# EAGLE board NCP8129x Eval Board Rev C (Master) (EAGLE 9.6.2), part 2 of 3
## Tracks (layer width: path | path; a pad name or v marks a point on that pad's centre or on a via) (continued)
VIN  (via drill 0.15 pad 0.3) (continued)
  other vias: 37.23,60.63 37.63,60.63 38.03,60.63 38.43,60.63 38.83,60.63 39.23,60.63 39.63,60.63 40.03,60.63 37.43,60.98 37.83,60.98 38.23,60.98 38.63,60.98 39.03,60.98 39.43,60.98 39.83,60.98 37.23,61.33 37.63,61.33 38.03,61.33 38.43,61.33 38.83,61.33 39.23,61.33 39.63,61.33 40.03,61.33 37.43,61.68 37.83,61.68 38.23,61.68 38.63,61.68 39.03,61.68 39.43,61.68 39.83,61.68 37.23,62.03 37.63,62.03 38.03,62.03 38.43,62.03 38.83,62.03 39.23,62.03 39.63,62.03 40.03,62.03 37.43,62.38 37.83,62.38 38.23,62.38 38.63,62.38 39.03,62.38 39.43,62.38 39.83,62.38 37.23,62.73 37.63,62.73 38.03,62.73 38.43,62.73 38.83,62.73 39.23,62.73 39.63,62.73 40.03,62.73 37.43,63.08 37.83,63.08 38.23,63.08 38.63,63.08 39.03,63.08 39.43,63.08 39.83,63.08 37.23,63.43 37.63,63.43 38.03,63.43 38.43,63.43 38.83,63.43 39.23,63.43 39.63,63.43 40.03,63.43 37.43,63.78 37.83,63.78 38.23,63.78 38.63,63.78 39.03,63.78 39.43,63.78 39.83,63.78 65.38,31.13 65.78,31.13 66.18,31.13 66.58,31.13 66.98,31.13 67.38,31.13 67.78,31.13 65.18,31.43 65.58,31.43 65.98,31.43 66.38,31.43 66.78,31.43 67.18,31.43 67.58,31.43 67.98,31.43 65.38,31.73 65.78,31.73 66.18,31.73 66.58,31.73 66.98,31.73 67.38,31.73 67.78,31.73 65.18,32.03 65.58,32.03 65.98,32.03 66.38,32.03 66.78,32.03 67.18,32.03 67.58,32.03 67.98,32.03 65.38,32.33 65.78,32.33 66.18,32.33 66.58,32.33 66.98,32.33 67.38,32.33 67.78,32.33 65.18,32.63 65.58,32.63 65.98,32.63 66.38,32.63 66.78,32.63 67.18,32.63 67.58,32.63 67.98,32.63 65.38,32.93 65.78,32.93 66.18,32.93 66.58,32.93 66.98,32.93 67.38,32.93 67.78,32.93 65.18,33.23 65.58,33.23 65.98,33.23 66.38,33.23 66.78,33.23 67.18,33.23 67.58,33.23 67.98,33.23 67.78,33.53 67.38,33.53 66.98,33.53 66.58,33.53 66.18,33.53 65.78,33.53 65.38,33.53 65.18,33.83 65.58,33.83 65.98,33.83 66.38,33.83 66.78,33.83 67.18,33.83 67.58,33.83 67.98,33.83 37.43,60.28 37.03,60.28 37.83,60.28 38.23,60.28 38.63,60.28 39.03,60.28 39.43,60.28 39.83,60.28 37.23,59.93 37.63,59.93 38.03,59.93 38.43,59.93 38.83,59.93 39.23,59.93 39.63,59.93 36.83,59.93 37.03,59.58 37.43,59.58 37.83,59.58 38.23,59.58 38.63,59.58 39.03,59.58 39.43,59.58 39.83,59.58 36.83,59.23 37.23,59.23 37.63,59.23 38.03,59.23 38.43,59.23 38.83,59.23 39.23,59.23 39.63,59.23 39.83,58.88 39.43,58.88 39.03,58.88 38.63,58.88 38.23,58.88 37.83,58.88 37.43,58.88 37.03,58.88 36.63,58.88 36.63,59.58 36.43,59.23 36.23,58.88 36.43,58.53 36.03,58.53 36.83,58.53 37.23,58.53 37.63,58.53 38.03,58.53 38.43,58.53 38.83,58.53 39.23,58.53 39.63,58.53 40.03,58.53 35.78,49.83 35.38,49.83 34.98,49.83 34.58,49.83 34.18,49.83 33.78,49.83 33.38,49.83 32.98,49.83 32.58,49.83 32.18,49.83 35.58,49.53 35.18,49.53 34.78,49.53 34.38,49.53 33.98,49.53 33.58,49.53 33.18,49.53 32.38,49.53 32.78,49.53 31.98,49.53 35.98,49.53 32.18,49.23 32.58,49.23 32.98,49.23 33.38,49.23 33.78,49.23 34.18,49.23 34.58,49.23 34.98,49.23 35.38,49.23 35.78,49.23 31.98,48.93 32.38,48.93 32.78,48.93 33.18,48.93 33.58,48.93 33.98,48.93 34.38,48.93 34.78,48.93 35.18,48.93 35.58,48.93 35.98,48.93 32.18,48.63 32.58,48.63 32.98,48.63 33.38,48.63 33.78,48.63 34.18,48.63 34.58,48.63 34.98,48.63 35.38,48.63 35.78,48.63 31.98,48.33 32.38,48.33 32.78,48.33 33.18,48.33 33.58,48.33 33.98,48.33 34.38,48.33 34.78,48.33 35.18,48.33 35.58,48.33 35.98,48.33 35.78,48.03 35.38,48.03 34.98,48.03 34.58,48.03 34.18,48.03 32.18,48.03 32.58,48.03 32.98,48.03 33.38,48.03 33.78,48.03 45.08,49.83 44.68,49.83 44.28,49.83 43.88,49.83 43.48,49.83 43.08,49.83 42.68,49.83 42.28,49.83 41.88,49.83 41.48,49.83 44.88,49.53 44.48,49.53 44.08,49.53 43.68,49.53 43.28,49.53 42.88,49.53 42.48,49.53 41.68,49.53 42.08,49.53 41.28,49.53 45.28,49.53 41.48,49.23 41.88,49.23 42.28,49.23 42.68,49.23 43.08,49.23 43.48,49.23 43.88,49.23 44.28,49.23 44.68,49.23 45.08,49.23 41.28,48.93 41.68,48.93 42.08,48.93 42.48,48.93 42.88,48.93 43.28,48.93 43.68,48.93 44.08,48.93 44.48,48.93 44.88,48.93 45.28,48.93 41.48,48.63 41.88,48.63 42.28,48.63 42.68,48.63 43.08,48.63 43.48,48.63 43.88,48.63 44.28,48.63 44.68,48.63 45.08,48.63 41.28,48.33 41.68,48.33 42.08,48.33 42.48,48.33 42.88,48.33 43.28,48.33 43.68,48.33 44.08,48.33 44.48,48.33 44.88,48.33 45.28,48.33 45.08,48.03 44.68,48.03 44.28,48.03 43.88,48.03 43.48,48.03 41.48,48.03 41.88,48.03 42.28,48.03 42.68,48.03 43.08,48.03 36.13,56.48 35.73,56.48 35.33,56.48 35.93,56.18 35.53,56.18 36.13,55.88 35.73,55.88 35.33,55.88 35.93,55.58 35.53,55.58 36.13,55.28 35.73,55.28 35.33,55.28 41.93,56.48 41.53,56.48 41.13,56.48 41.73,56.18 41.33,56.18 41.93,55.88 41.53,55.88 41.13,55.88 41.73,55.58 41.33,55.58 41.93,55.28 41.53,55.28 41.13,55.28 35.53,54.98 35.33,54.68 35.53,54.38 35.33,54.08 35.53,53.78 35.33,53.48 35.13,54.98 35.13,54.38 35.13,53.78 34.93,53.48 34.73,53.78 34.93,54.08 34.93,54.68 34.73,54.38 34.53,54.08 34.33,53.78 34.53,53.48 34.53,54.68 34.33,54.38 34.13,54.08 33.93,53.78 34.13,53.48 34.13,54.68 33.93,54.38 33.73,54.08 33.53,53.78 33.73,53.48 33.53,54.38 33.73,54.68 41.73,54.98 41.93,54.68 41.73,54.38 41.93,54.08 41.73,53.78 41.93,53.48 42.13,53.78 42.13,54.38 42.13,54.98 42.33,54.68 42.53,54.38 42.33,54.08 42.53,53.78 42.33,53.48 42.73,54.68 43.13,54.68 43.53,54.68 42.93,54.38 43.33,54.38 43.73,54.38 42.73,54.08 43.13,54.08 43.53,54.08 42.93,53.78 43.33,53.78 43.73,53.78 42.73,53.48 43.13,53.48 43.53,53.48 36.63,56.63 37.43,56.63 38.23,56.63 39.03,56.63 40.63,56.63 37.03,56.23 37.83,56.23 38.63,56.23 40.23,56.23 36.63,55.83 37.43,55.83 38.23,55.83 39.83,55.83 40.63,55.83 37.03,55.43 37.83,55.43 39.43,55.43 40.23,55.43 36.63,55.03 37.43,55.03 39.03,55.03 39.83,55.03 40.63,55.03 37.03,54.63 36.23,54.63 38.63,54.63 39.43,54.63 40.23,54.63 41.03,54.63 36.63,54.23 38.23,54.23 39.03,54.23 39.83,54.23 40.63,54.23 36.23,53.83 37.83,53.83 38.63,53.83 39.43,53.83 40.23,53.83 41.03,53.83 41.43,53.43 40.63,53.43 39.83,53.43 39.03,53.43 38.23,53.43 37.43,53.43 35.83,53.43 35.43,53.03 34.63,53.03 33.83,53.03 35.03,52.63 34.23,52.63 41.03,51.43 41.83,51.43 42.63,51.43 43.43,51.43 40.23,51.43 39.43,51.43 38.63,51.43 37.83,51.43 43.03,51.03 42.23,51.03 41.43,51.03 40.63,51.03 39.83,51.03 39.03,51.03 38.23,51.03 37.43,51.03 37.83,50.63 38.63,50.63 39.43,50.63 40.23,50.63 41.03,50.63 41.83,50.63 42.63,50.63 43.43,50.63 44.23,50.63 37.03,50.63 37.43,50.23 38.23,50.23 39.03,50.23 39.83,50.23 40.63,50.23 41.43,50.23 42.23,50.23 43.03,50.23 43.83,50.23 44.63,50.23 36.63,50.23 35.83,50.23 35.03,50.23 34.23,50.23 33.43,50.23 32.63,50.23 37.03,49.83 37.83,49.83 38.63,49.83 39.43,49.83 40.23,49.83 41.03,49.83 40.63,49.43 39.83,49.43 39.03,49.43 38.23,49.43 37.43,49.43 36.63,49.43 36.23,49.83 37.03,49.03 37.83,49.03 38.63,49.03 39.43,49.03 40.23,49.03 36.63,48.63 37.43,48.63 38.23,48.63 39.03,48.63 39.83,48.63 40.63,48.63 37.03,48.23 37.83,48.23 38.63,48.23 39.43,48.23 40.23,48.23 36.63,47.83 37.43,47.83 38.23,47.83 39.03,47.83 39.83,47.83 40.63,47.83 40.63,44.63 41.43,44.63 42.23,44.63 43.03,44.63 43.83,44.63 44.63,44.63 39.83,44.63 39.03,44.63 38.23,44.63 37.43,44.63 36.63,44.63 35.83,44.63 35.03,44.63 34.23,44.63 33.43,44.63 33.03,44.23 33.83,44.23 34.63,44.23 35.43,44.23 36.23,44.23 37.03,44.23 37.83,44.23 38.63,44.23 39.43,44.23 40.23,44.23 41.03,44.23 41.83,44.23 42.63,44.23 43.43,44.23 44.23,44.23 45.03,44.23 32.63,43.83 33.43,43.83 34.23,43.83 35.03,43.83 35.83,43.83 36.63,43.83 37.43,43.83 38.23,43.83 39.03,43.83 39.83,43.83 40.63,43.83 41.43,43.83 42.23,43.83 43.03,43.83 43.83,43.83 44.63,43.83 32.23,43.43 33.03,43.43 33.83,43.43 34.63,43.43 35.43,43.43 36.23,43.43 37.03,43.43 37.83,43.43 38.63,43.43 39.43,43.43 40.23,43.43 45.03,43.43 44.23,43.43 43.43,43.43 42.63,43.43 41.83,43.43 41.03,43.43 32.63,43.03 33.43,43.03 34.23,43.03 35.03,43.03 35.83,43.03 36.63,43.03 37.43,43.03 38.23,43.03 39.03,43.03 44.63,43.03 43.83,43.03 43.03,43.03 42.23,43.03 41.43,43.03 40.63,43.03 39.83,43.03 45.03,42.63 44.23,42.63 43.43,42.63 42.63,42.63 41.83,42.63 41.03,42.63 40.23,42.63 39.43,42.63 38.63,42.63 37.83,42.63 32.23,42.63 33.03,42.63 33.83,42.63 34.63,42.63 35.43,42.63 36.23,42.63 37.03,42.63 32.63,42.23 33.43,42.23 34.23,42.23 35.03,42.23 35.83,42.23 36.63,42.23 37.43,42.23 38.23,42.23 39.03,42.23 39.83,42.23 40.63,42.23 41.43,42.23 42.23,42.23 43.03,42.23 43.83,42.23 44.63,42.23 45.03,41.83 44.23,41.83 43.43,41.83 42.63,41.83 41.83,41.83 41.03,41.83 40.23,41.83 39.43,41.83 38.63,41.83 37.83,41.83 37.03,41.83 36.23,41.83 35.43,41.83 34.63,41.83 33.83,41.83 33.03,41.83 32.23,41.83 32.63,41.43 33.43,41.43 34.23,41.43 35.03,41.43 35.83,41.43 36.63,41.43 37.43,41.43 38.23,41.43 39.03,41.43 39.83,41.43 40.63,41.43 41.43,41.43 42.23,41.43 43.03,41.43 43.83,41.43 44.63,41.43 45.03,41.03 44.23,41.03 43.43,41.03 42.63,41.03 41.83,41.03 41.03,41.03 40.23,41.03 39.43,41.03 38.63,41.03 37.83,41.03 37.03,41.03 36.23,41.03 35.43,41.03 34.63,41.03 33.83,41.03 33.03,41.03 32.23,41.03 32.63,40.63 33.43,40.63 34.23,40.63 35.03,40.63 35.83,40.63 36.63,40.63 37.43,40.63 38.23,40.63 39.03,40.63 44.63,40.63 43.83,40.63 43.03,40.63 42.23,40.63 41.43,40.63 40.63,40.63 39.83,40.63 45.03,40.23 44.23,40.23 43.43,40.23 42.63,40.23 41.83,40.23 41.03,40.23 40.23,40.23 39.43,40.23 38.63,40.23 37.83,40.23 32.23,40.23 33.03,40.23 33.83,40.23 34.63,40.23 35.43,40.23 36.23,40.23 37.03,40.23 32.63,39.83 33.43,39.83 34.23,39.83 35.03,39.83 35.83,39.83 36.63,39.83 37.43,39.83 38.23,39.83 39.03,39.83 39.83,39.83 40.63,39.83 41.43,39.83 42.23,39.83 43.03,39.83 43.83,39.83 44.63,39.83 45.03,39.43 44.23,39.43 43.43,39.43 42.63,39.43 41.83,39.43 41.03,39.43 40.23,39.43 39.43,39.43 38.63,39.43 37.83,39.43 37.03,39.43 36.23,39.43 35.43,39.43 34.63,39.43 33.83,39.43 33.03,39.43 32.23,39.43 32.63,39.03 33.43,39.03 34.23,39.03 35.03,39.03 35.83,39.03 36.63,39.03 37.43,39.03 38.23,39.03 39.03,39.03 39.83,39.03 40.63,39.03 41.43,39.03 42.23,39.03 43.03,39.03 43.83,39.03 44.63,39.03 45.03,38.63 44.23,38.63 43.43,38.63 42.63,38.63 41.83,38.63 41.03,38.63 40.23,38.63 39.43,38.63 38.63,38.63 37.83,38.63 37.03,38.63 36.23,38.63 35.43,38.63 34.63,38.63 33.83,38.63 33.03,38.63 32.23,38.63 32.63,38.23 33.43,38.23 34.23,38.23 35.03,38.23 35.83,38.23 36.63,38.23 37.43,38.23 38.23,38.23 39.03,38.23 44.63,38.23 43.83,38.23 43.03,38.23 42.23,38.23 41.43,38.23 40.63,38.23 39.83,38.23 45.03,37.83 44.23,37.83 43.43,37.83 42.63,37.83 41.83,37.83 41.03,37.83 40.23,37.83 39.43,37.83 38.63,37.83 37.83,37.83 32.23,37.83 33.03,37.83 33.83,37.83 34.63,37.83 35.43,37.83 36.23,37.83 37.03,37.83 32.63,37.43 33.43,37.43 34.23,37.43 35.03,37.43 35.83,37.43 36.63,37.43 37.43,37.43 38.23,37.43 39.03,37.43 39.83,37.43 40.63,37.43 41.43,37.43 42.23,37.43 43.03,37.43 43.83,37.43 44.63,37.43 45.03,37.03 44.23,37.03 43.43,37.03 42.63,37.03 41.83,37.03 41.03,37.03 40.23,37.03 39.43,37.03 38.63,37.03 37.83,37.03 37.03,37.03 36.23,37.03 35.43,37.03 34.63,37.03 33.83,37.03 33.03,37.03 32.23,37.03 32.63,36.63 33.43,36.63 34.23,36.63 35.03,36.63 35.83,36.63 36.63,36.63 37.43,36.63 38.23,36.63 39.03,36.63 39.83,36.63 40.63,36.63 41.43,36.63 42.23,36.63 43.03,36.63 43.83,36.63 44.63,36.63 45.03,36.23 44.23,36.23 43.43,36.23 42.63,36.23 41.83,36.23 41.03,36.23 40.23,36.23 39.43,36.23 38.63,36.23 37.83,36.23 37.03,36.23 36.23,36.23 35.43,36.23 34.63,36.23 33.83,36.23 33.03,36.23 32.23,36.23 32.63,35.83 33.43,35.83 34.23,35.83 35.03,35.83 35.83,35.83 36.63,35.83 37.43,35.83 38.23,35.83 39.03,35.83 44.63,35.83 43.83,35.83 43.03,35.83 42.23,35.83 41.43,35.83 40.63,35.83 39.83,35.83 45.03,35.43 44.23,35.43 43.43,35.43 42.63,35.43 41.83,35.43 41.03,35.43 40.23,35.43 39.43,35.43 38.63,35.43 37.83,35.43 32.23,35.43 33.03,35.43 33.83,35.43 34.63,35.43 35.43,35.43 36.23,35.43 37.03,35.43 32.63,35.03 33.43,35.03 34.23,35.03 35.03,35.03 35.83,35.03 36.63,35.03 37.43,35.03 38.23,35.03 39.03,35.03 39.83,35.03 40.63,35.03 41.43,35.03 42.23,35.03 43.03,35.03 43.83,35.03 44.63,35.03 45.03,34.63 44.23,34.63 43.43,34.63 42.63,34.63 41.83,34.63 41.03,34.63 40.23,34.63 39.43,34.63 38.63,34.63 37.83,34.63 37.03,34.63 36.23,34.63 35.43,34.63 34.63,34.63 33.83,34.63 33.03,34.63 32.23,34.63 32.63,34.23 33.43,34.23 34.23,34.23 35.03,34.23 35.83,34.23 36.63,34.23 37.43,34.23 38.23,34.23 39.03,34.23 39.83,34.23 40.63,34.23 41.43,34.23 42.23,34.23 43.03,34.23 43.83,34.23 44.63,34.23 45.03,33.83 44.23,33.83 43.43,33.83 42.63,33.83 41.83,33.83 41.03,33.83 40.23,33.83 39.43,33.83 38.63,33.83 37.83,33.83 37.03,33.83 36.23,33.83 35.43,33.83 34.63,33.83 33.83,33.83 33.03,33.83 32.23,33.83 32.63,33.43 33.43,33.43 34.23,33.43 35.03,33.43 35.83,33.43 36.63,33.43 37.43,33.43 38.23,33.43 39.03,33.43 44.63,33.43 43.83,33.43 43.03,33.43 42.23,33.43 41.43,33.43 40.63,33.43 39.83,33.43 45.03,33.03 44.23,33.03 43.43,33.03 42.63,33.03 41.83,33.03 41.03,33.03 40.23,33.03 39.43,33.03 38.63,33.03 37.83,33.03 32.23,33.03 33.03,33.03 33.83,33.03 34.63,33.03 35.43,33.03 36.23,33.03 37.03,33.03 32.63,32.63 33.43,32.63 34.23,32.63 35.03,32.63 35.83,32.63 36.63,32.63 37.43,32.63 38.23,32.63 39.03,32.63 39.83,32.63 40.63,32.63 41.43,32.63 42.23,32.63 43.03,32.63 43.83,32.63 44.63,32.63 45.03,32.23 44.23,32.23 43.43,32.23 42.63,32.23 41.83,32.23 41.03,32.23 40.23,32.23 39.43,32.23 38.63,32.23 37.83,32.23 37.03,32.23 36.23,32.23 35.43,32.23 34.63,32.23 33.83,32.23 33.03,32.23 32.23,32.23 32.63,31.83 33.43,31.83 34.23,31.83 35.03,31.83 35.83,31.83 36.63,31.83 37.43,31.83 38.23,31.83 39.03,31.83 39.83,31.83 40.63,31.83 41.43,31.83 42.23,31.83 43.03,31.83 43.83,31.83 44.63,31.83 45.03,31.43 44.23,31.43 43.43,31.43 42.63,31.43 41.83,31.43 41.03,31.43 40.23,31.43 39.43,31.43 38.63,31.43 37.83,31.43 37.03,31.43 36.23,31.43 35.43,31.43 34.63,31.43 33.83,31.43 33.03,31.43 32.23,31.43 32.63,31.03 33.43,31.03 34.23,31.03 35.03,31.03 35.83,31.03 36.63,31.03 37.43,31.03 38.23,31.03 39.03,31.03 44.63,31.03 43.83,31.03 43.03,31.03 42.23,31.03 41.43,31.03 40.63,31.03 39.83,31.03 45.03,30.63 44.23,30.63 43.43,30.63 42.63,30.63 41.83,30.63 41.03,30.63 40.23,30.63 39.43,30.63 38.63,30.63 37.83,30.63 32.23,30.63 33.03,30.63 33.83,30.63 34.63,30.63 35.43,30.63 36.23,30.63 37.03,30.63 32.63,30.23 33.43,30.23 34.23,30.23 35.03,30.23 35.83,30.23 36.63,30.23 37.43,30.23 38.23,30.23 39.03,30.23 39.83,30.23 40.63,30.23 41.43,30.23 42.23,30.23 43.03,30.23 43.83,30.23 44.63,30.23 45.03,29.83 44.23,29.83 43.43,29.83 42.63,29.83 41.83,29.83 41.03,29.83 40.23,29.83 39.43,29.83 38.63,29.83 37.83,29.83 37.03,29.83 36.23,29.83 35.43,29.83 34.63,29.83 33.83,29.83 33.03,29.83 32.23,29.83 32.63,29.43 33.43,29.43 34.23,29.43 35.03,29.43 35.83,29.43 36.63,29.43 37.43,29.43 38.23,29.43 39.03,29.43 39.83,29.43 40.63,29.43 41.43,29.43 42.23,29.43 43.03,29.43 43.83,29.43 44.63,29.43 45.03,29.03 44.23,29.03 43.43,29.03 42.63,29.03 41.83,29.03 41.03,29.03 40.23,29.03 39.43,29.03 38.63,29.03 37.83,29.03 37.03,29.03 36.23,29.03 35.43,29.03 34.63,29.03 33.83,29.03 33.03,29.03 32.23,29.03 32.63,28.63 33.43,28.63 34.23,28.63 35.03,28.63 35.83,28.63 36.63,28.63 37.43,28.63 38.23,28.63 39.03,28.63 44.63,28.63 43.83,28.63 43.03,28.63 42.23,28.63 41.43,28.63 40.63,28.63 39.83,28.63 45.03,28.23 44.23,28.23 43.43,28.23 42.63,28.23 41.83,28.23 41.03,28.23 40.23,28.23 39.43,28.23 38.63,28.23 37.83,28.23 32.23,28.23 33.03,28.23 33.83,28.23 34.63,28.23 35.43,28.23 36.23,28.23 37.03,28.23 32.63,27.83 33.43,27.83 34.23,27.83 35.03,27.83 35.83,27.83 36.63,27.83 37.43,27.83 38.23,27.83 39.03,27.83 39.83,27.83 40.63,27.83 41.43,27.83 42.23,27.83 43.03,27.83 43.83,27.83 44.63,27.83 45.03,27.43 44.23,27.43 43.43,27.43 42.63,27.43 41.83,27.43 41.03,27.43 40.23,27.43 39.43,27.43 38.63,27.43 37.83,27.43 37.03,27.43 36.23,27.43 35.43,27.43 34.63,27.43 33.83,27.43 33.03,27.43 32.23,27.43 32.63,27.03 33.43,27.03 34.23,27.03 35.03,27.03 35.83,27.03 36.63,27.03 37.43,27.03 38.23,27.03 39.03,27.03 39.83,27.03 40.63,27.03 41.43,27.03 42.23,27.03 43.03,27.03 43.83,27.03 44.63,27.03 45.03,26.63 44.23,26.63 43.43,26.63 42.63,26.63 41.83,26.63 41.03,26.63 40.23,26.63 39.43,26.63 38.63,26.63 37.83,26.63 37.03,26.63 36.23,26.63 35.43,26.63 34.63,26.63 33.83,26.63 33.03,26.63 32.23,26.63 32.63,26.23 33.43,26.23 34.23,26.23 35.03,26.23 35.83,26.23 36.63,26.23 37.43,26.23 38.23,26.23 39.03,26.23 44.63,26.23 43.83,26.23 43.03,26.23 42.23,26.23 41.43,26.23 40.63,26.23 39.83,26.23 45.03,25.83 44.23,25.83 43.43,25.83 42.63,25.83 41.83,25.83 41.03,25.83 40.23,25.83 39.43,25.83 38.63,25.83 37.83,25.83 32.23,25.83 33.03,25.83 33.83,25.83 34.63,25.83 35.43,25.83 36.23,25.83 37.03,25.83 32.63,25.43 33.43,25.43 34.23,25.43 35.03,25.43 35.83,25.43 36.63,25.43 37.43,25.43 38.23,25.43 39.03,25.43 39.83,25.43 40.63,25.43 41.43,25.43 42.23,25.43 43.03,25.43 43.83,25.43 44.63,25.43 45.03,25.03 44.23,25.03 43.43,25.03 42.63,25.03 41.83,25.03 41.03,25.03 40.23,25.03 39.43,25.03 38.63,25.03 37.83,25.03 37.03,25.03 36.23,25.03 35.43,25.03 34.63,25.03 33.83,25.03 33.03,25.03 33.43,24.63 34.23,24.63 35.03,24.63 35.83,24.63 36.63,24.63 37.43,24.63 38.23,24.63 39.03,24.63 39.83,24.63 40.63,24.63 41.43,24.63 42.23,24.63 43.03,24.63 43.83,24.63 44.63,24.63 45.03,24.23 44.23,24.23 43.43,24.23 42.63,24.23 41.83,24.23 41.03,24.23 40.23,24.23 39.43,24.23 38.63,24.23 37.83,24.23 37.03,24.23 36.23,24.23 35.43,24.23 34.63,24.23 33.83,24.23 45.43,39.83 45.43,39.03 45.43,38.23 45.43,37.43 45.43,36.63 45.43,35.83 45.43,35.03 45.43,34.23 45.43,33.43 45.43,32.63 45.43,31.83 45.43,31.03 45.83,31.43 45.83,32.23 45.83,33.03 45.83,33.83 45.83,34.63 45.83,35.43 45.83,36.23 45.83,37.03 45.83,37.83 45.83,38.63 45.83,39.43 46.23,39.03 46.23,38.23 46.23,37.43 46.23,36.63 46.23,35.83 46.23,35.03 46.23,34.23 46.23,33.43 46.23,32.63 46.23,31.83 46.63,32.23 46.63,33.03 46.63,33.83 46.63,34.63 46.63,35.43 46.63,36.23 46.63,37.03 46.63,37.83 46.63,38.63 47.03,38.23 47.03,37.43 47.03,36.63 47.03,35.83 47.03,35.03 47.03,34.23 47.03,33.43 47.03,32.63 47.43,33.03 47.43,33.83 47.43,34.63 47.43,35.43 47.43,36.23 47.43,37.03 47.43,37.83 47.83,36.63 47.83,37.43 47.83,35.83 47.83,35.03 47.83,34.23 47.83,33.43 48.23,33.83 48.23,34.63 48.23,35.43 48.23,36.23 48.23,37.03 48.23,33.03 47.83,32.63 48.23,32.23 47.83,31.83 48.23,31.43 47.83,31.03 48.23,30.63 47.83,30.23 48.23,29.83 47.83,29.43 48.23,29.03 47.83,28.63 48.23,28.23 47.83,27.83 48.23,27.43 47.83,27.03 47.43,32.23 47.43,31.43 47.43,30.63 47.43,29.83 47.43,29.03 47.43,28.23 47.43,27.43 47.03,27.83 47.03,28.63 47.03,29.43 47.03,30.23 47.03,31.03 47.03,31.83 46.63,31.43 46.63,30.63 46.63,29.83 46.63,29.03 46.63,28.23 46.23,29.43 46.23,30.23 46.23,31.03 45.83,30.63 45.83,29.83 46.23,28.63 45.83,29.03 45.43,30.23 45.43,29.43 45.43,28.63 45.83,28.23 46.23,27.83 46.63,27.43 47.03,27.03 47.43,26.63 47.83,26.23 48.23,26.63 45.43,27.83 45.83,27.43 46.23,27.03 46.63,26.63 47.03,26.23 47.43,25.83 47.83,25.43 48.23,25.83 48.23,25.03 45.43,27.03 45.83,26.63 46.23,26.23 46.63,25.83 47.03,25.43 47.43,25.03 47.83,24.63 48.23,24.23 45.43,26.23 45.83,25.83 46.23,25.43 46.63,25.03 47.03,24.63 47.43,24.23 47.83,23.83 48.23,23.43 45.43,25.43 45.83,25.03 46.23,24.63 46.63,24.23 47.03,23.83 47.43,23.43 47.83,23.03 48.23,22.63 45.43,24.63 45.83,24.23 46.23,23.83 46.63,23.43 47.03,23.03 47.43,22.63 47.83,22.23 48.23,21.83 48.63,23.83 49.43,23.83 50.23,23.83 51.03,23.83 51.83,23.83 52.63,23.83 53.43,23.83 54.23,23.83 55.03,23.83 55.83,23.83 56.63,23.83 57.43,23.83 58.23,23.83 59.03,23.83 59.83,23.83 60.63,23.83 61.43,23.83 61.03,23.43 60.23,23.43 59.43,23.43 58.63,23.43 57.83,23.43 57.03,23.43 56.23,23.43 55.43,23.43 54.63,23.43 53.83,23.43 53.03,23.43 52.23,23.43 51.43,23.43 49.03,23.43 49.83,23.43 50.63,23.43 48.63,23.03 49.43,23.03 50.23,23.03 51.03,23.03 51.83,23.03 52.63,23.03 53.43,23.03 54.23,23.03 55.03,23.03 55.83,23.03 60.63,23.03 59.83,23.03 59.03,23.03 58.23,23.03 57.43,23.03 56.63,23.03 49.03,22.63 49.83,22.63 50.63,22.63 51.43,22.63 52.23,22.63 53.03,22.63 53.83,22.63 54.63,22.63 55.43,22.63 56.23,22.63 57.03,22.63 57.83,22.63 58.63,22.63 59.43,22.63 60.23,22.63 61.03,22.63 60.63,22.23 60.23,21.83 34.23,23.83 35.03,23.83 35.83,23.83 36.63,23.83 37.43,23.83 38.23,23.83 39.03,23.83 39.83,23.83 40.63,23.83 41.43,23.83 42.23,23.83 43.03,23.83 43.83,23.83 44.63,23.83 45.43,23.83 34.63,23.43 35.43,23.43 36.23,23.43 37.03,23.43 37.83,23.43 38.63,23.43 39.43,23.43 40.23,23.43 41.03,23.43 41.83,23.43 42.63,23.43 43.43,23.43 44.23,23.43 45.03,23.43 45.83,23.43 35.03,23.03 35.83,23.03 36.63,23.03 37.43,23.03 38.23,23.03 39.03,23.03 39.83,23.03 40.63,23.03 41.43,23.03 42.23,23.03 43.03,23.03 43.83,23.03 44.63,23.03 45.43,23.03 46.23,23.03 35.43,22.63 36.23,22.63 37.03,22.63 37.83,22.63 38.63,22.63 39.43,22.63 40.23,22.63 41.03,22.63 41.83,22.63 42.63,22.63 43.43,22.63 44.23,22.63 45.03,22.63 45.83,22.63 46.63,22.63 35.83,22.23 36.63,22.23 37.43,22.23 38.23,22.23 39.03,22.23 39.83,22.23 40.63,22.23 41.43,22.23 42.23,22.23 43.03,22.23 43.83,22.23 44.63,22.23 45.43,22.23 46.23,22.23 47.03,22.23 36.23,21.83 37.03,21.83 37.83,21.83 38.63,21.83 39.43,21.83 40.23,21.83 41.03,21.83 41.83,21.83 42.63,21.83 43.43,21.83 44.23,21.83 45.03,21.83 45.83,21.83 46.63,21.83 47.43,21.83 48.63,22.23 49.03,21.83 49.43,22.23 49.83,21.83 50.23,22.23 50.63,21.83 51.03,22.23 51.43,21.83 51.83,22.23 52.23,21.83 52.63,22.23 53.03,21.83 53.43,22.23 53.83,21.83 54.23,22.23 54.63,21.83 55.03,22.23 55.43,21.83 55.83,22.23 56.23,21.83 56.63,22.23 57.03,21.83 57.43,22.23 57.83,21.83 58.23,22.23 58.63,21.83 59.03,22.23 59.43,21.83 59.83,22.23 36.63,21.43 37.43,21.43 38.23,21.43 39.03,21.43 39.83,21.43 40.63,21.43 41.43,21.43 42.23,21.43 43.03,21.43 59.83,21.43 59.03,21.43 58.23,21.43 57.43,21.43 56.63,21.43 55.83,21.43 55.03,21.43 54.23,21.43 53.43,21.43 52.63,21.43 51.83,21.43 51.03,21.43 50.23,21.43 49.43,21.43 48.63,21.43 47.83,21.43 47.03,21.43 46.23,21.43 45.43,21.43 44.63,21.43 43.83,21.43 37.03,21.03 37.83,21.03 38.63,21.03 39.43,21.03 40.23,21.03 41.03,21.03 41.83,21.03 42.63,21.03 43.43,21.03 44.23,21.03 45.03,21.03 45.83,21.03 46.63,21.03 47.43,21.03 48.23,21.03 49.03,21.03 49.83,21.03 50.63,21.03 51.43,21.03 52.23,21.03 53.03,21.03 53.83,21.03 54.63,21.03 55.43,21.03 56.23,21.03 57.03,21.03 57.83,21.03 58.63,21.03 59.43,21.03 37.43,20.63 38.23,20.63 39.03,20.63 39.83,20.63 40.63,20.63 41.43,20.63 42.23,20.63 43.03,20.63 43.83,20.63 44.63,20.63 45.43,20.63 46.23,20.63 47.03,20.63 47.83,20.63 48.63,20.63 49.43,20.63 50.23,20.63 51.03,20.63 51.83,20.63 52.63,20.63 53.43,20.63 54.23,20.63 55.03,20.63 55.83,20.63 56.63,20.63 57.43,20.63 58.23,20.63 59.03,20.63 37.83,20.23 38.63,20.23 39.43,20.23 40.23,20.23 41.03,20.23 41.83,20.23 42.63,20.23 43.43,20.23 44.23,20.23 45.03,20.23 45.83,20.23 46.63,20.23 47.43,20.23 48.23,20.23 49.03,20.23 49.83,20.23 50.63,20.23 51.43,20.23 52.23,20.23 53.03,20.23 53.83,20.23 54.63,20.23 55.43,20.23 56.23,20.23 57.03,20.23 57.83,20.23 58.63,20.23 38.23,19.83 39.03,19.83 39.83,19.83 40.63,19.83 41.43,19.83 42.23,19.83 43.03,19.83 43.83,19.83 44.63,19.83 45.43,19.83 46.23,19.83 47.03,19.83 47.83,19.83 48.63,19.83 49.43,19.83 50.23,19.83 51.03,19.83 51.83,19.83 52.63,19.83 53.43,19.83 54.23,19.83 55.03,19.83 55.83,19.83 56.63,19.83 57.43,19.83 58.23,19.83 38.63,19.43 39.43,19.43 40.23,19.43 41.03,19.43 41.83,19.43 42.63,19.43 43.43,19.43 44.23,19.43 45.03,19.43 45.83,19.43 46.63,19.43 47.43,19.43 48.23,19.43 49.03,19.43 49.83,19.43 50.63,19.43 51.43,19.43 52.23,19.43 53.03,19.43 53.83,19.43 54.63,19.43 55.43,19.43 56.23,19.43 57.03,19.43 57.83,19.43 39.03,19.03 39.83,19.03 40.63,19.03 41.43,19.03 42.23,19.03 43.03,19.03 43.83,19.03 44.63,19.03 45.43,19.03 46.23,19.03 47.03,19.03 47.83,19.03 48.63,19.03 49.43,19.03 50.23,19.03 51.03,19.03 51.83,19.03 52.63,19.03 53.43,19.03 54.23,19.03 55.03,19.03 55.83,19.03 56.63,19.03 57.43,19.03 57.03,18.63 56.23,18.63 55.43,18.63 54.63,18.63 53.83,18.63 53.03,18.63 52.23,18.63 51.43,18.63 50.63,18.63 49.83,18.63 49.03,18.63 48.23,18.63 47.43,18.63 46.63,18.63 39.43,18.63 40.23,18.63 41.03,18.63 41.83,18.63 42.63,18.63 43.43,18.63 44.23,18.63 45.03,18.63 45.83,18.63 39.83,18.23 40.63,18.23 41.43,18.23 42.23,18.23 43.03,18.23 43.83,18.23 44.63,18.23 45.43,18.23 46.23,18.23 47.03,18.23 47.83,18.23 48.63,18.23 49.43,18.23 50.23,18.23 51.03,18.23 51.83,18.23 52.63,18.23 53.43,18.23 54.23,18.23 55.03,18.23 55.83,18.23 56.63,18.23 56.23,17.83 55.43,17.83 54.63,17.83 53.83,17.83 53.03,17.83 52.23,17.83 51.43,17.83 50.63,17.83 49.83,17.83 49.03,17.83 48.23,17.83 47.43,17.83 46.63,17.83 45.83,17.83 45.03,17.83 44.23,17.83 43.43,17.83 42.63,17.83 41.83,17.83 41.03,17.83 40.23,17.83 40.63,17.43 41.43,17.43 42.23,17.43 43.03,17.43 43.83,17.43 44.63,17.43 45.43,17.43 46.23,17.43 47.03,17.43 47.83,17.43 48.63,17.43 49.43,17.43 50.23,17.43 51.03,17.43 51.83,17.43 52.63,17.43 53.43,17.43 54.23,17.43 55.03,17.43 55.83,17.43 55.43,17.03 54.63,17.03 53.83,17.03 53.03,17.03 52.23,17.03 51.43,17.03 50.63,17.03 49.83,17.03 49.03,17.03 48.23,17.03 47.43,17.03 46.63,17.03 45.83,17.03 45.03,17.03 44.23,17.03 43.43,17.03 42.63,17.03 41.83,17.03 41.03,17.03 41.43,16.63 42.23,16.63 43.03,16.63 43.83,16.63 44.63,16.63 45.43,16.63 46.23,16.63 47.03,16.63 47.83,16.63 48.63,16.63 49.43,16.63 50.23,16.63 51.03,16.63 51.83,16.63 52.63,16.63 53.43,16.63 54.23,16.63 55.03,16.63 54.63,16.23 53.83,16.23 53.03,16.23 52.23,16.23 51.43,16.23 50.63,16.23 49.83,16.23 49.03,16.23 48.23,16.23 47.43,16.23 46.63,16.23 45.83,16.23 45.03,16.23 44.23,16.23 43.43,16.23 42.63,16.23 41.83,16.23 42.23,15.83 43.03,15.83 43.83,15.83 44.63,15.83 45.43,15.83 46.23,15.83 47.03,15.83 47.83,15.83 48.63,15.83 49.43,15.83 50.23,15.83 51.03,15.83 51.83,15.83 52.63,15.83 53.43,15.83 54.23,15.83 53.83,15.43 53.03,15.43 52.23,15.43 51.43,15.43 50.63,15.43 49.83,15.43 49.03,15.43 48.23,15.43 47.43,15.43 46.63,15.43 45.83,15.43 45.03,15.43 44.23,15.43 43.43,15.43 42.63,15.43 43.03,15.03 43.83,15.03 44.63,15.03 45.43,15.03 46.23,15.03 47.03,15.03 47.83,15.03 48.63,15.03 49.43,15.03 50.23,15.03 51.03,15.03 51.83,15.03 52.63,15.03 53.43,15.03 53.83,14.63 53.03,14.63 52.23,14.63 51.43,14.63 50.63,14.63 49.83,14.63 49.03,14.63 48.23,14.63 47.43,14.63 46.63,14.63 45.83,14.63 45.03,14.63 44.23,14.63 43.43,14.63 43.83,14.23 44.63,14.23 45.43,14.23 46.23,14.23 47.03,14.23 47.83,14.23 48.63,14.23 49.43,14.23 50.23,14.23 51.03,14.23 51.83,14.23 52.63,14.23 53.43,14.23 53.83,13.83 53.43,13.43 53.83,13.03 53.43,12.63 53.83,12.23 53.43,11.83 53.83,11.43 53.43,11.03 53.83,10.63 53.43,10.23 53.83,9.83 53.43,9.43 53.83,9.03 53.43,8.63 53.83,8.23 53.43,7.83 53.83,7.43 53.43,7.03 53.83,6.63 53.43,6.23 53.83,5.83 53.43,5.43 53.83,5.03 53.43,4.63 53.83,4.23 53.43,3.83 53.83,3.43 53.43,3.03 53.03,3.43 52.63,3.03 52.23,3.43 51.83,3.03 51.43,3.43 51.03,3.03 50.63,3.43 50.23,3.03 49.83,3.43 49.43,3.03 49.03,3.43 48.63,3.03 48.23,3.43 47.83,3.03 47.43,3.43 47.03,3.03 46.63,3.43 46.23,3.03 45.83,3.43 45.43,3.03 45.03,3.43 44.63,3.03 44.23,3.43 43.83,3.03 43.83,3.83 44.23,4.23 43.83,4.63 44.23,5.03 43.83,5.43 44.23,5.83 43.83,6.23 44.23,6.63 43.83,7.03 44.23,7.43 43.83,7.83 44.23,8.23 43.83,8.63 44.23,9.03 43.83,9.43 44.23,9.83 43.83,10.23 44.23,10.63 43.83,11.03 44.23,11.43 43.83,11.83 44.23,12.23 43.83,12.63 44.23,13.03 43.83,13.43 44.23,13.83 44.63,13.43 44.63,12.63 44.63,11.83 44.63,11.03 44.63,10.23 44.63,9.43 44.63,8.63 44.63,3.83 44.63,4.63 44.63,5.43 44.63,6.23 44.63,7.03 44.63,7.83 53.03,4.23 53.03,5.03 53.03,5.83 53.03,6.63 53.03,7.43 53.03,8.23 53.03,9.03 53.03,13.83 53.03,13.03 53.03,12.23 53.03,11.43 53.03,10.63 53.03,9.83 68.18,31.73 68.18,32.33 68.38,32.03 68.58,31.73 68.38,31.43 68.18,31.13 68.78,31.43 68.58,31.13 68.98,31.13 68.78,30.83 69.18,30.83 68.38,30.83 68.98,30.53 69.38,30.53 68.58,30.53 69.18,30.23 69.58,30.23 69.38,29.93 68.78,30.23 68.98,29.93 69.18,29.63 69.58,29.63 68.78,29.63 68.98,29.33 69.38,29.33 69.18,29.03 69.58,29.03 68.58,29.33 68.78,29.03 69.38,28.73 68.98,28.73 69.18,28.43 69.58,28.43 68.78,28.43 68.58,28.73 68.38,28.43 68.38,29.03 68.38,29.63 68.58,29.93 68.38,30.23 68.18,30.53 68.18,29.93 67.98,30.83 67.98,30.23 67.78,30.53 67.58,30.83 68.18,32.93 68.18,33.53 68.38,33.23 68.58,32.93 68.38,32.63 68.78,32.63 68.58,32.33 68.98,32.33 69.38,32.33 68.78,32.03 69.18,32.03 69.18,32.63 68.98,31.73 69.38,31.73 69.58,32.03 69.18,31.43 69.58,31.43 69.38,31.13 69.58,30.83 67.18,30.83
  pour +5V (no thermals): 40.33,63.93 36.93,63.93 36.93,60.53 36.93,60.18 36.23,59.48 35.63,58.88 35.63,58.43 40.18,58.43 40.18,58.73 39.98,58.93 39.98,60.38 40.13,60.53 40.33,60.53
  pour GND (no thermals): 36.93,63.93 36.93,60.18 36.58,59.83 35.63,58.88 35.63,58.43 40.18,58.43 40.18,58.73 39.98,58.93 39.98,60.38 40.03,60.43 40.13,60.53 40.33,60.53 40.33,63.93
  pour Top (no thermals): 36.93,63.93 36.93,60.53 36.93,60.33 36.78,60.18 36.78,60.03 35.98,59.23 33.28,59.23 33.18,59.23 33.18,58.68 35.18,56.68 35.18,55.23 35.18,55.18 34.98,54.98 34.78,54.78 34.53,54.78 33.58,54.78 33.48,54.68 33.43,54.63 33.43,54.38 33.43,51.48 31.88,49.93 31.88,25.88 43.48,14.28 43.48,2.58 54.23,2.58 54.23,15.58 61.63,22.98 61.63,36.98 48.68,36.98 47.38,38.28 45.43,40.23 45.43,49.58 45.43,49.78 45.08,50.13 43.83,51.38 43.83,54.38 43.83,54.63 43.73,54.73 43.68,54.78 43.53,54.78 42.53,54.78 42.23,55.08 42.08,55.23 42.08,55.53 42.08,56.83 39.98,58.93 39.98,60.38 40.08,60.48 40.13,60.53 40.33,60.53 40.33,63.93
  pour Bottom (no thermals): 36.93,63.93 36.93,60.33 36.78,60.18 36.78,60.08 36.78,60.03 36.58,59.83 35.23,58.48 35.23,56.43 35.23,55.63 33.43,55.63 33.43,53.33 33.43,51.48 32.43,50.48 31.88,49.93 31.88,49.83 31.88,25.88 42.93,14.83 43.48,14.28 43.48,2.58 54.23,2.58 54.23,15.58 61.58,22.93 61.63,22.98 61.63,23.13 61.63,36.98 48.68,36.98 48.08,37.58 45.43,40.23 45.43,49.53 45.43,49.78 45.23,49.98 43.83,51.38 43.83,55.63 42.08,55.63 42.08,56.58 44.13,58.63 44.13,59.23 43.28,59.23 43.03,58.98 42.28,58.98 40.18,58.98 39.98,59.18 39.98,60.38 40.03,60.43 40.13,60.53 40.33,60.53 40.33,63.93
  pour Power/fusetofuse1 (isolate 0.3, no thermals): 75.43,63.93 -0.72,63.93 -0.72,0.03 75.43,0.03
  pour Power1 (isolate 0.3, no thermals): -0.72,63.93 -0.72,0.03 75.43,0.03 75.43,63.93
  pour Power/fusetoio1 (isolate 0.3, no thermals): -0.72,63.93 -0.72,0.03 75.43,0.03 75.43,63.93
  pour Power2 (isolate 0.3, no thermals): -0.72,63.93 -0.72,0.03 75.43,0.03 75.43,63.93
  pour Power/fusetoio2 (isolate 0.3, no thermals): -0.72,63.93 -0.72,0.03 75.43,0.03 75.43,63.93
  pour Power3 (isolate 0.3, no thermals): -0.72,63.93 -0.72,0.03 75.43,0.03 75.43,63.93
  pour Power/misc (isolate 0.3, no thermals): -0.72,63.93 -0.72,0.03 75.43,0.03 75.43,63.93
  pour Power4 (isolate 0.3, no thermals): -0.72,63.93 -0.72,0.03 75.43,0.03 75.43,63.93
  pour Bottom (no thermals): 61.28,36.98 61.58,36.98 64.63,33.93 66.28,33.93 68.13,33.93 68.58,33.48 69.73,32.33 69.73,30.08 69.73,28.18 68.28,28.18 68.28,29.18 68.28,29.48 67.93,29.83 66.78,30.98 65.43,30.98 63.83,30.98 61.63,28.78 61.28,29.13
VIN_S  (via drill 0.15 pad 0.3)  (1 unrouted)
  Power/fusetoio2 0.3: IC2.9 43.13,57.03 44.28,57.03 44.98,56.33 44.98,52.18 47.98,49.18 47.98,39.08 48.63,38.43 62.58,38.43 63.03,37.98 63.03,35.03 62.98,34.98 62.98,22.68 60.18,19.88 v60.18,8.83
  other vias: 40.38,59.78
VINF1  (via drill 0.15 pad 0.3)  (2 unrouted)
  Top 0.3: IC1.7 35.47,60.98 34.9,60.41 R1.1
  Top 0.5: R1.1 33.09,60.41 32.36,59.69 C9.1
  Power/fusetoio1 0.3: v14.48,47.63 20.18,47.63 25.28,52.73 31.18,52.73 32.33,53.88 v32.33,59.73
VINF2  (via drill 0.15 pad 0.3)  (2 unrouted)
  Power/fusetoio2 0.3: v14.48,78.08 9.73,78.08 5.98,81.83 5.98,96.58 7.33,97.93 30.03,97.93 47.93,80.03 47.93,75.23 50.88,72.28 50.88,61.18 49.48,59.78 v44.93,59.78
  Bottom 0.3: IC2.7 41.8,60.98 42.36,60.41 R2.1
  Bottom 0.5: R2.1 44.38,60.41 45.1,59.69 C10.1
VOUT  (via drill 0.15 pad 0.3)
